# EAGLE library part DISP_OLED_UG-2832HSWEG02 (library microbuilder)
128x32 I2C 0.91" Monochrome OLED Display
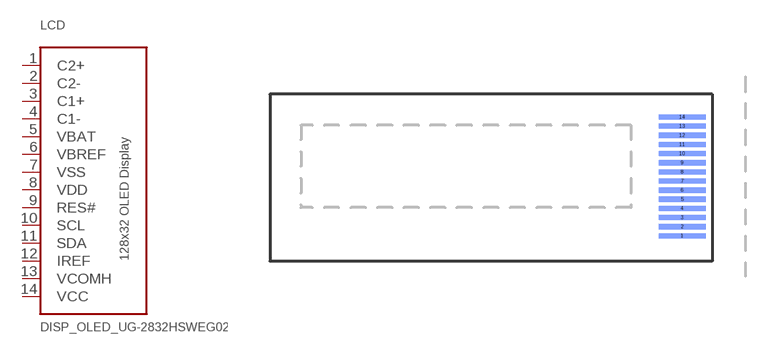
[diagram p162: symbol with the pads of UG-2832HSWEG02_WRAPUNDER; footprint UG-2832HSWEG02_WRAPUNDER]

Designator prefix LCD

## DISP_OLED_UG-2832HSWEG02  [UG-2832HSWEG02_WRAPUNDER]
1  C2+
2  C2-
3  C1+
4  C1-
5  VBAT  pwr
6  VBREF  pwr
7  VSS  pwr
8  VDD  pwr
9  RES#
10  SCL
11  SDA
12  IREF
13  VCOMH  pwr
14  VCC  pwr

## Footprint UG-2832HSWEG02_WRAPUNDER (pad centres in mm)
smd 3.2 x 0.35 bottom: 1 -2.03,-4.03; 2 -2.03,-3.41; 3 -2.03,-2.79; 4 -2.03,-2.17; 5 -2.03,-1.55; 6 -2.03,-0.93; 7 -2.03,-0.31; 8 -2.03,0.31; 9 -2.03,0.93; 10 -2.03,1.55; 11 -2.03,2.17; 12 -2.03,2.79; 13 -2.03,3.41; 14 -2.03,4.03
